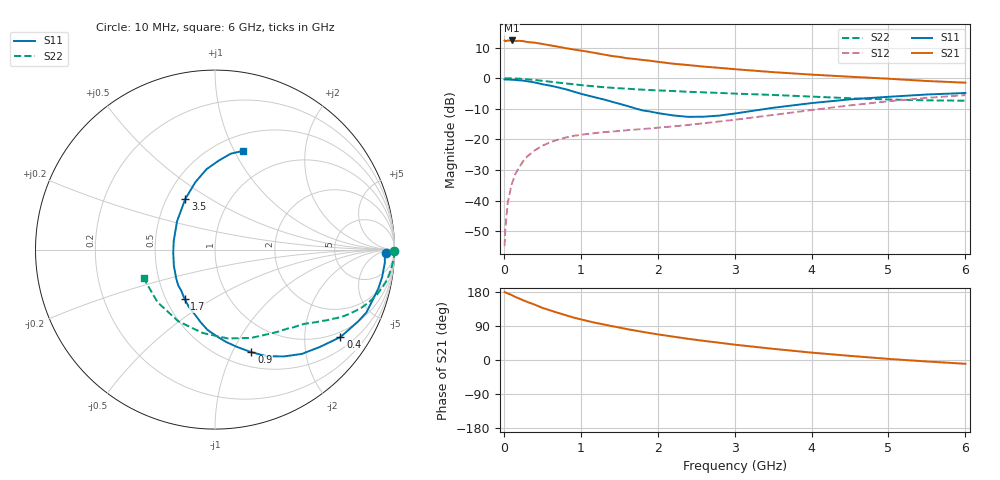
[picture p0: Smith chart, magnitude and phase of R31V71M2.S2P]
! SIEMENS Small Signal Semiconductors
! BFR181
! Si NPN RF Bipolar Junction Transistor in SOT23
! VCE = 1.75 V  IC = 1.2 mA
! Common Emitter S-Parameters:  May  1996
# GHz  S  MA  R  50
!  f  S11  S21  S12  S22
! GHz  MAG  ANG  MAG  ANG  MAG  ANG  MAG  ANG
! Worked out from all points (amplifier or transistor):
!   36 points, 10 MHz to 6 GHz, reference 50 ohm
!   highest |S21| = 12.3 dB at 100 MHz (marker M1)
!   |S21| within 3 dB of that: start of sweep to 924.4 MHz
!   unconditionally stable (mu >= 1): 1.875 GHz to 3.638 GHz
!   at 250 MHz: K = 0.17, MSG = 19.6 dB, |S12| = -27.2 dB
!   at 1.4 GHz: K = 0.83, MSG = 12.4 dB, |S12| = -17.5 dB
!   at 6 GHz: K = 0.88, MSG = 2.0 dB, |S12| = -5.5 dB
!   S11 on the Smith chart (normalised r, x): 10 MHz: 38, -14; 400 MHz: 0.83, -2.97; 900 MHz: 0.66, -1.19; 1.7 GHz: 0.62, -0.38; 3.5 GHz: 0.62, +0.39; 6 GHz: 0.66, +1.09
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0.01  0.9544 -1.0  4.125 179.4  0.0018 93.9  0.9988 -0.4
0.02  0.9468 -1.6  4.024 178.2  0.0035 92.3  0.9962 -0.9
0.05  0.949 -4.4  4.112 175.7  0.0091 87.4  0.9979 -2.1
0.1  0.9438 -9.2  4.132 171.6  0.0181 82.9  0.993 -4.2
0.15  0.9357 -13.3  4.037 166.4  0.0272 81.3  0.9867 -6.3
0.2  0.9225 -17.7  4.071 162.2  0.0352 78.7  0.9796 -8.3
0.25  0.9135 -22.5  4.032 157.8  0.0438 75.5  0.9705 -10.4
0.3  0.892 -26.7  3.903 153.6  0.052 73.4  0.9596 -12.2
0.4  0.852 -34.9  3.8 146.2  0.066 68.7  0.9353 -15.7
0.5  0.7964 -43.0  3.628 137.7  0.0786 64.1  0.9059 -18.9
0.6  0.7563 -50.2  3.442 131.1  0.0896 60.4  0.8763 -21.8
0.7  0.7094 -57.0  3.274 124.7  0.0988 57.1  0.8476 -24.1
0.9  0.6064 -70.5  2.959 112.3  0.1139 51.8  0.7975 -28.1
1.1  0.5178 -83.2  2.701 102.4  0.1233 48.4  0.7496 -31.3
1.4  0.4138 -101.0  2.308 89.5  0.134 45.9  0.6976 -35.3
1.7  0.3234 -121.6  2.059 78.0  0.1442 45.6  0.66 -38.5
2.2  0.2463 -158.5  1.723 61.7  0.1628 47.3  0.6166 -44.5
2.8  0.2445 154.2  1.476 45.6  0.1961 50.6  0.5737 -53.2
3.5  0.3279 120.2  1.255 29.5  0.2505 51.1  0.5319 -67.6
4.5  0.4505 96.0  1.056 10.9  0.3598 45.2  0.4697 -98.4
5.5  0.5413 80.7  0.899 -3.9  0.4769 32.7  0.4342 -137.6
6  0.5723 74.1  0.844 -10.0  0.5287 25.0  0.4283 -158.1
